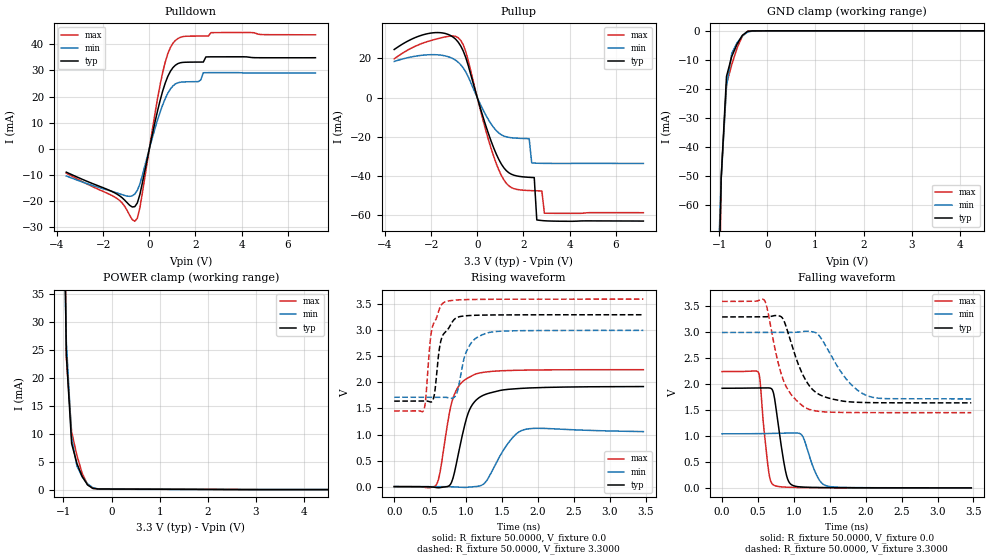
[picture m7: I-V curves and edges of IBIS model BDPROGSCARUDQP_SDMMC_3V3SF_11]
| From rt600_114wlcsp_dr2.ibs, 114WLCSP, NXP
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[Model] BDPROGSCARUDQP_SDMMC_3V3SF_11
|   Model BDPROGSCARUDQP_SDMMC_3V3SF_11
| This model was characterised for following simulation conditions:
| External (pad) voltage:
|   - Typ: 3.3V,   - Min: 3.0V,   - Max: 3.6V
| Library cells for typ/min/max conditions are connected as defined below:
|  IO - External Pad
|  A - Core Input
|  EN - Output Buffer Enable
|  ASRCN3V3[0] - REFH3V3 gnde REFH3V3
|  ASRCN3V3[1] - REFH3V3 REFH3V3 gnde
|  ASRCN3V3[2] - gnde
|  ASRCN3V3[3] - gnde REFH3V3 gnde
|  ASRCP3V3[0] - vdde3v3 vdde3v3 REFL3V3
|  ASRCP3V3[1] - vdde3v3 REFL3V3 vdde3v3
|  ASRCP3V3[2] - REFL3V3 vdde3v3 vdde3v3
|  ASRCP3V3[3] - REFL3V3 REFL3V3 vdde3v3
|  IOGC - NC
|  PDRV - vdd
|  PSW - vdd
|  REFH3V3 - REFH3V3
|  REFL3V3 - REFL3V3
|  ZI - NC
|  gnd - gnd
|  gnde - gnde
|  vdd - vdd
|  vdde3v3 - vdde3v3
| All other pins connected to ground
Model_type I/O
Polarity   Non-Inverting
Enable   Active-Low
Vinl =   0.7500V
Vinh =   2.2500V
Vmeas =  1.6500V
Cref =   30.0000pF
Rref =   1.0000M
Vref =   3.3000V
C_comp   2.1236pF   2.1099pF   2.1437pF
|C_comp_pullup   0.3619pF   0.3760pF   0.3515pF
|C_comp_pulldown   0.6265pF   0.6611pF   0.5987pF
[Model Spec]
| variable   typ   min   max
Vinh   2.0625V   1.8750V   2.2500V
Vinl   0.8250V   0.7500V   0.9000V
[Temperature Range]   25.0000   0.1250k   -40.0000
[Voltage Range]   3.3000V   3.0000V   3.6000V
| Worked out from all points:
|   slope of the pulldown table from 0 to 0.495 V, typ, clamps not added: 25.5 ohm
|   slope of the pullup table from 0 to 0.495 V, typ, clamps not added: 26.4 ohm
|   GND clamp passes 1 mA (typ) near -0.48 V on its own axis
|   POWER clamp passes 1 mA (typ) near -0.51 V on its own axis
|   rising waveform, R_fixture 50.0000, V_fixture 0.0: 20-80 % time 215ps typ, 264ps min, 187ps max; typ from 0 V to 1.92 V
|   rising waveform, R_fixture 50.0000, V_fixture 3.3000: 20-80 % time 135ps typ, 161ps min, 113ps max; typ from 1.64 V to 3.3 V
|   falling waveform, R_fixture 50.0000, V_fixture 0.0: 20-80 % time 124ps typ, 163ps min, 91.3ps max; typ from 1.92 V to 0 V
|   falling waveform, R_fixture 50.0000, V_fixture 3.3000: 20-80 % time 290ps typ, 371ps min, 253ps max; typ from 3.3 V to 1.64 V
[Pulldown]
|Voltage   I(typ)   I(min)   I(max)
-3.6V     -8.96mA    -10.4mA    -9.312mA
-1.4V     -17.38mA   -16.93mA   -19.05mA
-630mV    -22.15mA   -17.34mA   -27.77mA
-410mV    -17.5mA    -13.49mA   -22.58mA
250mV     10.41mA    7.919mA    13.77mA
580mV     22.14mA    16.85mA    29.29mA
800mV     27.69mA    21.24mA    36.37mA
1.13V     32mA       24.83mA    41.48mA
2.12V     33.19mA    25.7mA     43.14mA
2.34V     33.2mA     29.1mA     43.14mA
2.45V     35.15mA    29.12mA    43.15mA
7.2V      34.85mA    28.98mA    43.63mA
[Pullup]
|Voltage   I(typ)   I(min)   I(max)
-3.6V     24.55mA    18.43mA    19.79mA
-1.93V    33.06mA    21.91mA    29.4mA
-830mV    28.38mA    18.1mA     30.59mA
-500mV    20.5mA     13.11mA    23.56mA
1.04V     -33.9mA    -19mA      -39.66mA
2.25V     -40.75mA   -20.98mA   -47.5mA
2.36V     -40.82mA   -33.39mA   -47.55mA
2.47V     -40.88mA   -33.47mA   -47.6mA
2.58V     -62.51mA   -33.53mA   -47.64mA
2.8V      -62.83mA   -33.6mA    -47.71mA
2.91V     -62.93mA   -33.62mA   -59.07mA
7.2V      -63.09mA   -33.66mA   -58.81mA
[GND_clamp]
|Voltage   I(typ)   I(min)   I(max)
-3.6V     -5.131A    -2.875A    -8.762A
-1.07V    -134.2mA   -102.6mA   -176.8mA
-960mV    -50.84mA   -50.99mA   -50.43mA
-850mV    -15.74mA   -19.19mA   -18.44mA
-740mV    -8.808mA   -7.773mA   -11.63mA
-630mV    -4.596mA   -4.129mA   -5.959mA
-520mV    -1.551mA   -1.768mA   -1.8mA
-410mV    -182.3uA   -416.9uA   -135.3uA
-190mV    -16.94uA   -14.45uA   -23.35uA
7.2V      0A         0A         0A
[POWER_clamp]
|Voltage   I(typ)   I(min)   I(max)
-3.6V     5.01A      2.759A     8.682A
-1.05V    90.64mA    70.4mA     118.9mA
-940mV    24.29mA    26.42mA    23.58mA
-830mV    8.246mA    9.229mA    10.3mA
-720mV    4.663mA    4.226mA    6.11mA
-610mV    2.344mA    2.293mA    2.91mA
-500mV    850.8uA    1.048mA    919.3uA
-390mV    222uA      361.4uA    219.3uA
-280mV    111uA      115.7uA    149.6uA
-60mV     99.3uA     71.05uA    139.3uA
7.2V      0A         0A         0A
[Ramp]
| variable   typ   min   max
dV/dt_r  1.1521/0.2146n   0.6335/0.2637n   1.3463/0.1866n
dV/dt_f  0.9946/0.2895n   0.7688/0.3709n   1.2879/0.2530n
R_load = 50.0000
[Rising Waveform]
R_fixture= 50.0000
V_fixture= 0.0
V_fixture_min= 0.0
V_fixture_max= 0.0
|time   V(typ)   V(min)   V(max)
0s        169.4uV    152.5uV    200.5uV
585.5ps   -18.23mV   217uV      33.44mV
639.8ps   -18.78mV   171.6uV    287.1mV
775.8ps   30.64mV    -2.041mV   1.464V
899.1ps   665.2mV    -11.76mV   1.93V
1.014ns   1.345V     -12.83mV   2.076V
1.114ns   1.62V      -1.371mV   2.149V
1.264ns   1.767V     74.71mV    2.198V
1.8ns     1.888V     1.089V     2.235V
3.47ns    1.92V      1.056V     2.244V
[Rising Waveform]
R_fixture= 50.0000
V_fixture= 3.3000
V_fixture_min= 3.0000
V_fixture_max= 3.6000
|time   V(typ)   V(min)   V(max)
0s        1.641V     1.716V     1.451V
409.3ps   1.643V     1.716V     1.463V
524.4ps   1.631V     1.716V     3.019V
565.1ps   1.817V     1.716V     3.171V
640.1ps   2.737V     1.717V     3.447V
710ps     2.962V     1.715V     3.546V
851.9ps   3.227V     1.738V     3.58V
1.018ns   3.28V      2.628V     3.59V
1.272ns   3.293V     2.939V     3.594V
3.47ns    3.298V     2.998V     3.598V
[Falling Waveform]
R_fixture= 50.0000
V_fixture= 0.0
V_fixture_min= 0.0
V_fixture_max= 0.0
|time   V(typ)   V(min)   V(max)
0s        1.922V     1.043V     2.244V
508.3ps   1.929V     1.047V     2.218V
646.6ps   1.929V     1.049V     332.5mV
725.8ps   1.761V     1.051V     47.2mV
881.9ps   329.9mV    1.056V     14.31mV
984.3ps   46.68mV    1.06V      9.168mV
1.121ns   15.23mV    997.1mV    5.626mV
1.318ns   7.249mV    240.1mV    2.997mV
1.462ns   4.875mV    36.32mV    1.969mV
3.47ns    189.6uV    365.8uV    202.6uV
[Falling Waveform]
R_fixture= 50.0000
V_fixture= 3.3000
V_fixture_min= 3.0000
V_fixture_max= 3.6000
|time   V(typ)   V(min)   V(max)
0s        3.298V     2.998V     3.598V
589.5ps   3.301V     2.998V     3.617V
774.9ps   3.323V     3V         2.444V
859.9ps   3.228V     3V         2.053V
1.04ns    2.463V     3.002V     1.682V
1.175ns   2.053V     3.024V     1.536V
1.343ns   1.81V      2.951V     1.477V
1.727ns   1.666V     2.103V     1.454V
2.005ns   1.646V     1.787V     1.452V
3.47ns    1.641V     1.717V     1.451V
